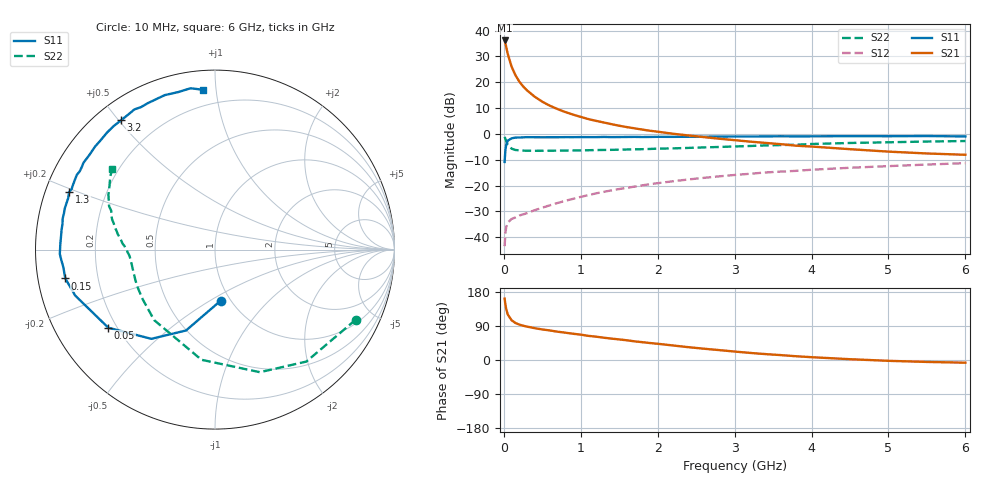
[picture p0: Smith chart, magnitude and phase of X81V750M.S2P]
! SIEMENS Small Signal Semiconductors
! BFP136W
! Si NPN RF Bipolar Junction Transistor in SOT343
! VCE = 1.75 V  IC = 50 mA
! Common Emitter S-Parameters:  September  1994
# GHz  S  MA  R  50
!  f  S11  S21  S12  S22
! GHz  MAG  ANG  MAG  ANG  MAG  ANG  MAG  ANG
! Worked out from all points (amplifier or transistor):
!   40 points, 10 MHz to 6 GHz, reference 50 ohm
!   highest |S21| = 36.2 dB at 10 MHz (marker M1)
!   |S21| within 3 dB of that: start of sweep to 34.42 MHz
!   unconditionally stable (mu >= 1): 588.8 MHz to 2.86 GHz
!   at 200 MHz: K = 0.56, MSG = 25.9 dB, |S12| = -31.6 dB
!   at 1.5 GHz: K = 1.12, MAG = 10.1 dB, |S12| = -21.4 dB
!   at 6 GHz: K = 0.98, MSG = 1.6 dB, |S12| = -11.3 dB
!   S11 on the Smith chart (normalised r, x): 10 MHz: 0.90, -0.56; 50 MHz: 0.17, -0.32; 150 MHz: 0.08, -0.09; 1.3 GHz: 0.07, +0.19; 3.2 GHz: 0.07, +0.51; 6 GHz: 0.10, +0.92
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0.01  0.2866 -83.7  64.5 162.1  0.0067 70.8  0.8759 -26.5
0.02  0.4785 -109.7  56.67 146.7  0.0119 58.8  0.8051 -50.8
0.03  0.6107 -125.5  48.93 135.2  0.0155 51.0  0.7273 -69.9
0.05  0.7368 -143.8  35.81 120.5  0.0192 38.1  0.6185 -97.0
0.1  0.8199 -161.8  20.16 104.9  0.0225 31.3  0.5189 -130.8
0.15  0.8494 -169.1  13.77 97.8  0.0241 32.2  0.4886 -145.7
0.2  0.8507 -173.4  10.35 93.6  0.0263 34.3  0.4795 -153.9
0.25  0.8588 -176.3  8.352 90.5  0.0276 36.4  0.4751 -159.1
0.3  0.8649 -178.4  6.991 88.2  0.0292 38.8  0.4718 -162.6
0.4  0.8623 177.8  5.266 84.0  0.0333 44.0  0.4709 -167.1
0.5  0.861 175.0  4.201 80.6  0.0372 47.5  0.4713 -170.1
0.6  0.8618 172.9  3.503 77.9  0.0415 50.2  0.4725 -172.1
0.7  0.862 170.3  3.019 74.6  0.046 53.0  0.4741 -173.4
0.9  0.8654 166.6  2.362 69.3  0.0553 55.5  0.4775 -175.8
1.1  0.8667 162.1  1.933 63.7  0.0652 57.2  0.4833 -177.4
1.3  0.8738 158.5  1.662 58.8  0.0755 57.8  0.4892 -178.9
1.7  0.8751 151.6  1.281 49.2  0.0954 57.0  0.503 178.1
2.2  0.8762 143.2  1.007 38.3  0.121 54.3  0.5247 174.5
3.2  0.8908 126.0  0.709 18.7  0.1692 45.8  0.5833 165.4
4.5  0.9051 108.0  0.506 2.1  0.221 33.7  0.6676 152.8
5.5  0.9092 98.6  0.418 -5.1  0.255 25.7  0.7118 145.1
6  0.893 94.3  0.394 -7.1  0.2717 21.3  0.728 141.8
